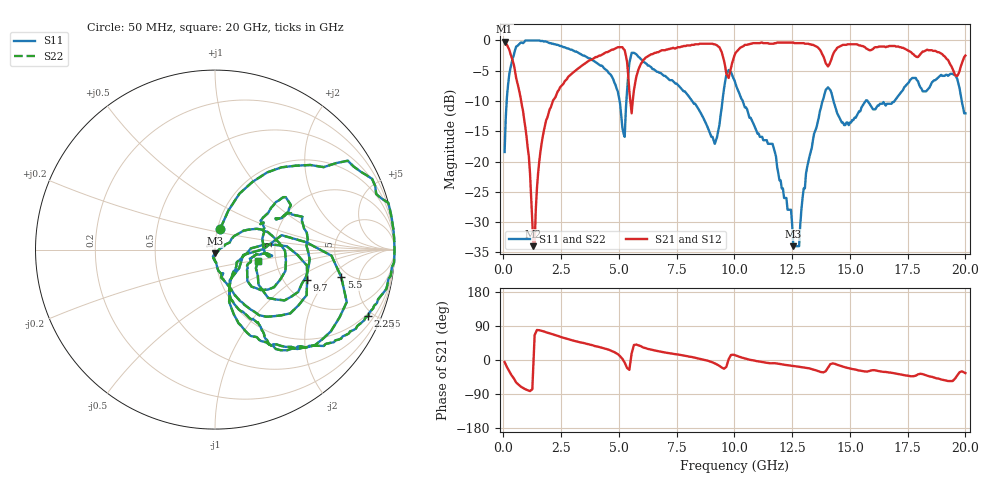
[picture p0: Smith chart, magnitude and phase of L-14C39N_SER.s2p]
# MHZ S MA R 50
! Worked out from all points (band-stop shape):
!   400 points, 50 MHz to 20 GHz, reference 50 ohm
!   highest |S21| = -0.18 dB at 50 MHz (marker M1); lowest = -34.0 dB at 1.3 GHz (marker M2)
!   |S21| within 3 dB of the highest: 9.944 GHz to 13.91 GHz (3.962 GHz wide, 33.2 % of centre); 14.19 GHz to 19.23 GHz (5.039 GHz wide, 30.1 % of centre)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
!   lowest |S11| = -34.0 dB at 12.55 GHz (marker M3), VSWR 1.04, Z = 49.8 - j1.98 ohm
!   |S11| at or under -10 dB: 8.169 GHz to 9.481 GHz (1.313 GHz wide, 14.9 % of centre); 10.36 GHz to 13.82 GHz (3.457 GHz wide, 28.6 % of centre); 14.29 GHz to 15.68 GHz (1.392 GHz wide, 9.29 % of centre)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
!   |S22| runs from -34.0 to 0.0 dB; largest |S21 - S12| = 0
!   S11 on the Smith chart (normalised r, x): 50 MHz: 1.03, +0.24; 2.25 GHz: 0.86, -4.68; 5.5 GHz: 4.32, -2.75; 9.7 GHz: 2.67, -1.27; 20 GHz: 1.62, -0.23
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50  0.12 75.9  0.98 -5.5  0.98 -5.5  0.12 75.9
400  0.71 41.6  0.68 -44.4  0.68 -44.4  0.71 41.6
1100  1 9.8  0.11 -81.0  0.11 -81.0  1 9.8
1300  1 3.5  0.02 -5.5  0.02 -5.5  1 3.5
1650  0.99 -7.2  0.14 77.1  0.14 77.1  0.99 -7.2
2250  0.93 -23.4  0.34 65.3  0.34 65.3  0.93 -23.4
3400  0.76 -44.8  0.62 45.7  0.62 45.7  0.76 -44.8
4750  0.48 -69.7  0.84 22.3  0.84 22.3  0.48 -69.7
5250  0.16 -10.9  0.83 -7.0  0.83 -7.0  0.16 -10.9
5500  0.72 -12.3  0.31 -4.3  0.31 -4.3  0.72 -12.3
5750  0.77 -43.9  0.5 40.7  0.5 40.7  0.77 -43.9
6700  0.55 -60.0  0.8 23.0  0.8 23.0  0.55 -60.0
9150  0.14 -30.0  0.93 -8.8  0.93 -8.8  0.14 -30.0
9700  0.54 -18.1  0.51 -8.1  0.51 -8.1  0.54 -18.1
10050  0.44 -56.1  0.79 12.3  0.79 12.3  0.44 -56.1
11650  0.14 -75.3  0.94 -8.4  0.94 -8.4  0.14 -75.3
12550  0.02 -95.6  0.96 -15.9  0.96 -15.9  0.02 -95.6
13350  0.13 35.2  0.92 -24.2  0.92 -24.2  0.13 35.2
14050  0.41 -16.8  0.61 -20.3  0.61 -20.3  0.41 -16.8
16700  0.3 31.3  0.9 -32.8  0.9 -32.8  0.3 31.3
19450  0.53 -16.1  0.58 -55.5  0.58 -55.5  0.53 -16.1
20000  0.25 -15.2  0.75 -34.6  0.75 -34.6  0.25 -15.2
